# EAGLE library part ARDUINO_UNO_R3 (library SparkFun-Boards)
Arduino R3 Footprint with SPI header Arduino Uno R3 Compatible Footprint. Matches PCB size of the original board. SparkFun Products: SAMD21 Dev Breakout RedBoard R3 Stackable Headers
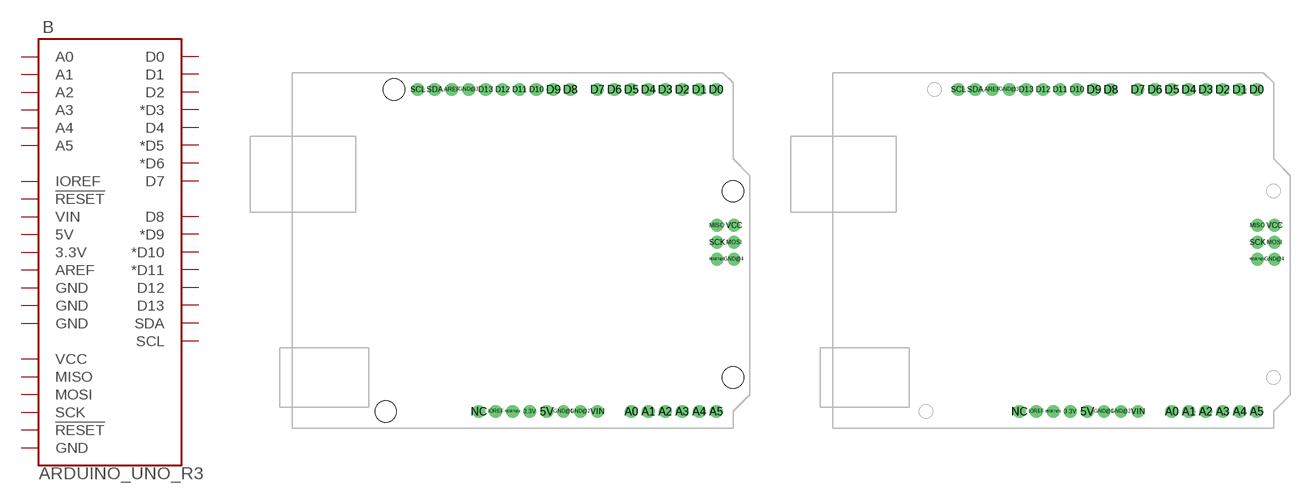
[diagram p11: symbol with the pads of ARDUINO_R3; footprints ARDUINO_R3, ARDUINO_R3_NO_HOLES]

Designator prefix B

## ARDUINO_UNO_R3  [ARDUINO_R3]
3.3V  3.3V
5V  5V
A0  A0
A1  A1
A2  A2
A3  A3
A4  A4
A5  A5
AREF  AREF
D0  D0
D1  D1
D2  D2
D3  *D3
D4  D4
D5  *D5
D6  *D6
D7  D7
D8  D8
D9  *D9
D10  *D10
D11  *D11
D12  D12
D13  D13
GND@1  GND
GND@2  GND
GND@3  GND
GND@4  GND
IOREF  IOREF
MISO  MISO
MOSI  MOSI
RESET@1  !RESET!
RESET@2  !RESET!
SCK  SCK
SCL  SCL
SDA  SDA
VCC  VCC
VIN  VIN

## ARDUINO_UNO_R3NO_HOLES  [ARDUINO_R3_NO_HOLES]
Pads as for ARDUINO_R3

## Footprint ARDUINO_R3 (pad centres in mm)
Arduino Uno R3 Footprint Includes mounting holes, and holes for ICSP header Specifications: Pin count: 38 Area:2.7x2.1in Datasheet referenced for footprint: Example device(s): Arduino Uno R3
drill 1.016 pad 1.93: 3.3V 2.54,-24.13; 5V 5.08,-24.13; A0 17.78,-24.13; A1 20.32,-24.13; A2 22.86,-24.13; A3 25.4,-24.13; A4 27.94,-24.13; A5 30.48,-24.13; AREF -9.144,24.13; D0 30.48,24.13; D1 27.94,24.13; D2 25.4,24.13; D3 22.86,24.13; D4 20.32,24.13; D5 17.78,24.13; D6 15.24,24.13; D7 12.7,24.13; D8 8.636,24.13; D9 6.096,24.13; D10 3.556,24.13; D11 1.016,24.13; D12 -1.524,24.13; D13 -4.064,24.13; GND@1 7.62,-24.13; GND@2 10.16,-24.13; GND@3 -6.604,24.13; GND@4 33.16,-1.32; IOREF -2.54,-24.13; MISO 30.62,3.76; MOSI 33.16,1.22; NC -5.08,-24.13; RESET@1 0,-24.13; RESET@2 30.62,-1.32; SCK 30.62,1.22; SCL -14.224,24.13; SDA -11.684,24.13; VCC 33.16,3.76; VIN 12.7,-24.13
hole 3.175 at -17.78,24.13
hole 3.175 at 33.02,8.89
hole 3.175 at 33.02,-19.05
hole 3.175 at -19.05,-24.13

## Footprint ARDUINO_R3_NO_HOLES (pad centres in mm)
Arduino Uno R3 Footprint Includes holes for ICSP header Specifications: Pin count: 38 Area:2.7x2.1in Example device(s): Arduino Uno R3
drill 1.016 pad 1.93: 3.3V 1.27,-24.13; 5V 3.81,-24.13; A0 16.51,-24.13; A1 19.05,-24.13; A2 21.59,-24.13; A3 24.13,-24.13; A4 26.67,-24.13; A5 29.21,-24.13; AREF -10.414,24.13; D0 29.21,24.13; D1 26.67,24.13; D2 24.13,24.13; D3 21.59,24.13; D4 19.05,24.13; D5 16.51,24.13; D6 13.97,24.13; D7 11.43,24.13; D8 7.366,24.13; D9 4.826,24.13; D10 2.286,24.13; D11 -0.254,24.13; D12 -2.794,24.13; D13 -5.334,24.13; GND@1 6.35,-24.13; GND@2 8.89,-24.13; GND@3 -7.874,24.13; GND@4 31.89,-1.32; IOREF -3.81,-24.13; MISO 29.35,3.76; MOSI 31.89,1.22; NC -6.35,-24.13; RESET@1 -1.27,-24.13; RESET@2 29.35,-1.32; SCK 29.35,1.22; SCL -15.494,24.13; SDA -12.954,24.13; VCC 31.89,3.76; VIN 11.43,-24.13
